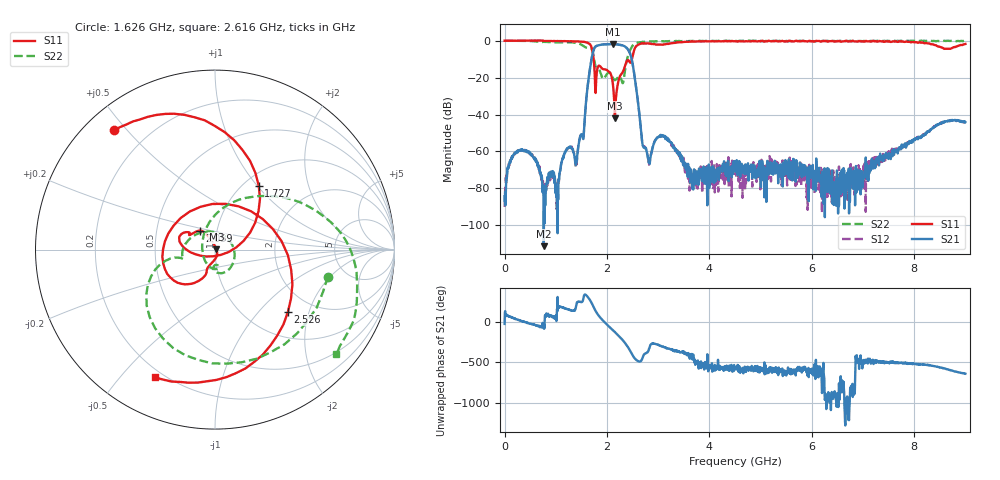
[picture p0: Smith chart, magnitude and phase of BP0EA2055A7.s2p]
!Agilent Technologies,E8358A,US40260310,A.06.04.32
!Agilent E8358A: A.06.04.32
!Date: Friday, May 08, 2020 03:22:50
!Correction: S11(Full 2 Port(1,2)) S21(Full 2 Port(1,2)) S12(Full 2 Port(1,2)) S22(Full 2 Port(1,2))
!S2P File: Measurements: S11, S21, S12, S22:
# Hz S  dB  R 50
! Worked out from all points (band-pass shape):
!   1601 points, 300 kHz to 9 GHz, reference 50 ohm
!   highest |S21| = -1.86 dB at 2.11 GHz (marker M1); lowest = -111.3 dB at 765.3 MHz (marker M2)
!   |S21| within 3 dB of the highest: 1.741 GHz to 2.411 GHz (670.3 MHz wide, 32.3 % of centre)
!   lowest |S11| = -42.0 dB at 2.155 GHz (marker M3), VSWR 1.02, Z = 50.8 + j0.138 ohm
!   |S11| at or under -10 dB: 1.739 GHz to 2.486 GHz (747.4 MHz wide, 35.4 % of centre)
!   |S22| runs from -23.1 to 0.1 dB; largest |S21 - S12| = 0.0095
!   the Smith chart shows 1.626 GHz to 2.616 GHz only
!   S11 on the Smith chart (normalised r, x): 1.626 GHz: 0.08, +0.46; 1.727 GHz: 1.16, +1.02; 2.059 GHz: 0.83, +0.18; 2.526 GHz: 1.51, -1.47; 2.616 GHz: 0.17, -0.62
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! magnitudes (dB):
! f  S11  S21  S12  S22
! 300 kHz  0.0  -84.3  -90.1  0.0
! 326.5 MHz  0.0  -59.4  -59.5  0.0
! 765.3 MHz  -0.2  -111.3  -77.6  -0.6
! 1.03 GHz  -0.2  -83.8  -99.4  -0.9
! 1.193 GHz  -0.3  -59.5  -60.0  -0.9
! 1.39 GHz  -0.4  -67.4  -68.9  -1.2
! 1.502 GHz  -0.6  -50.7  -50.8  -2.2
! 1.626 GHz  -1.2  -23.8  -23.7  -3.8
! 1.727 GHz  -7.3  -6.1  -6.1  -6.8
! 2.059 GHz  -17.3  -1.9  -1.9  -17.4
! 2.11 GHz  -22.3  -1.9  -1.8  -19.8
! 2.155 GHz  -42.0  -1.9  -1.9  -21.3
! 2.526 GHz  -5.4  -16.9  -16.8  -1.9
! 2.616 GHz  -2.1  -35.7  -35.6  -1.0
! 2.807 GHz  -1.5  -63.7  -64.3  -0.5
! 3.004 GHz  -2.2  -52.0  -52.6  -0.4
! 3.707 GHz  -0.5  -71.4  -71.8  -0.2
! 4.5 GHz  -0.3  -66.5  -68.5  -0.2
! 6.002 GHz  -0.2  -69.0  -69.7  -0.4
! 6.694 GHz  -0.4  -71.5  -86.2  -0.1
! 7.504 GHz  -0.4  -60.9  -59.8  -0.2
! 9 GHz  -1.8  -44.1  -44.0  -0.1
